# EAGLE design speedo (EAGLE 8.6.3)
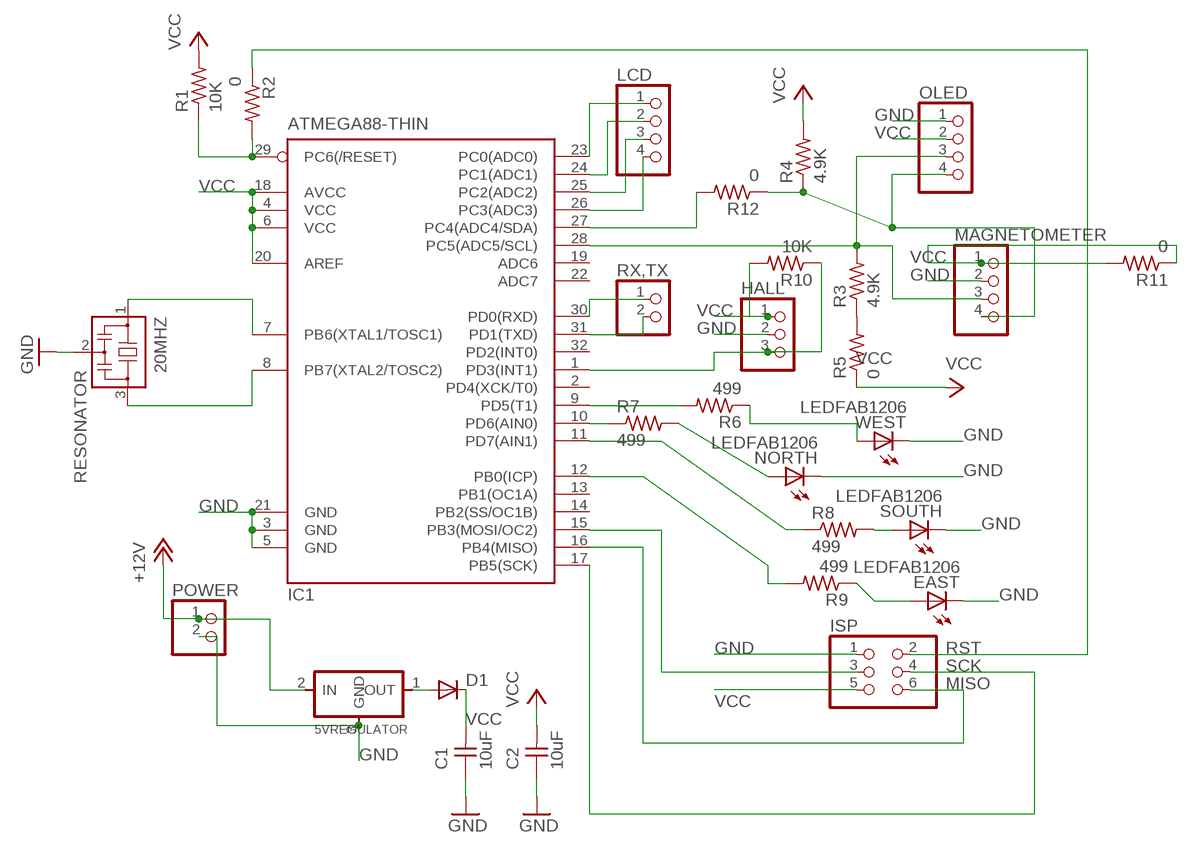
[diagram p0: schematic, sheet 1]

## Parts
5VREGULATOR  REGULATORSOT23  [SOT23]
20MHZ  RESONATOR  [EFOBM]
C1  10uF  CAP-UNPOLARIZEDFAB  [C1206FAB]
C2  10uF  CAP-UNPOLARIZEDFAB  [C1206FAB]
D1  DIODESOD123  [SOD123]
EAST  LEDFAB1206  [LED1206FAB]
HALL  PINHD-1X3  [1X03]
IC1  ATMEGA88-THIN  [TQFP32-08THIN]
ISP  PINHD-2X3-SMD  [2X03SMD]
LCD  PINHD-1X4  [1X04]
MAGNETOMETER  PINHD-1X4  [1X04]
NORTH  LEDFAB1206  [LED1206FAB]
OLED  PINHD-1X4  [1X04]
POWER  PINHD-1X2  [1X02]
R1  10K  RES-US1206FAB  [R1206FAB]
R2  0  RES-US1206FAB  [R1206FAB]
R3  4.9K  RES-US1206FAB  [R1206FAB]
R4  4.9K  RES-US1206FAB  [R1206FAB]
R5  0  RES-US1206FAB  [R1206FAB]
R6  499  RES-US1206FAB  [R1206FAB]
R7  499  RES-US1206FAB  [R1206FAB]
R8  499  RES-US1206FAB  [R1206FAB]
R9  499  RES-US1206FAB  [R1206FAB]
R10  10K  RES-US1206FAB  [R1206FAB]
R11  0  RES-US1206FAB  [R1206FAB]
R12  0  RES-US1206FAB  [R1206FAB]
RX,TX  PINHD-1X2  [1X02]
SOUTH  LEDFAB1206  [LED1206FAB]
WEST  LEDFAB1206  [LED1206FAB]

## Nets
+12V: 5VREGULATOR.2(IN) POWER.1
GND: 5VREGULATOR.3(GND) 20MHZ.2 C1.1 C2.1 EAST.2(C) HALL.2 IC1.3(GND) IC1.5(GND) IC1.21(GND) ISP.1 MAGNETOMETER.2 NORTH.2(C) OLED.1 POWER.2 SOUTH.2(C) WEST.2(C)
MISO: IC1.16(PB4(MISO)) ISP.6
N$1: IC1.29(PC6(/RESET)) R1.1 R2.2
N$2: 20MHZ.1 IC1.7(PB6(XTAL1/TOSC1))
N$3: 20MHZ.3 IC1.8(PB7(XTAL2/TOSC2))
N$4: 5VREGULATOR.1(OUT) D1.ANODE(A)
N$5: HALL.3 IC1.1(PD3(INT1)) R10.1
N$6: IC1.30(PD0(RXD)) RX,TX.1
N$7: MAGNETOMETER.4 OLED.4 R4.1 R12.1
N$8: IC1.28(PC5(ADC5/SCL)) MAGNETOMETER.3 OLED.3 R3.2
N$9: IC1.31(PD1(TXD)) RX,TX.2
N$10: IC1.27(PC4(ADC4/SDA)) R12.2
N$11: EAST.1(A) R9.1
N$12: IC1.9(PD5(T1)) R6.2
N$13: R6.1 WEST.1(A)
N$14: IC1.23(PC0(ADC0)) LCD.1
N$15: IC1.24(PC1(ADC1)) LCD.2
N$16: IC1.25(PC2(ADC2)) LCD.3
N$17: IC1.15(PB3(MOSI/OC2)) ISP.3
N$18: IC1.26(PC3(ADC3)) LCD.4
N$19: NORTH.1(A) R7.2
N$20: R8.2 SOUTH.1(A)
N$21: IC1.12(PB0(ICP)) R9.2
N$22: IC1.10(PD6(AIN0)) R7.1
N$23: IC1.11(PD7(AIN1)) R8.1
RST: ISP.2 R2.1
SCK: IC1.17(PB5(SCK)) ISP.4
VCC: C1.2 C2.2 D1.CATHODE(C) HALL.1 IC1.4(VCC) IC1.6(VCC) IC1.18(AVCC) IC1.20(AREF) ISP.5 MAGNETOMETER.1 OLED.2 R1.2 R3.1 R4.2 R5.1 R5.2 R10.2 R11.1 R11.2
Unconnected: IC1.2(PD4(XCK/T0)) IC1.13(PB1(OC1A)) IC1.14(PB2(SS/OC1B)) IC1.19(ADC6) IC1.22(ADC7) IC1.32(PD2(INT0))

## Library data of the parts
5VREGULATOR = fab:REGULATOR
20MHZ = fab:RESONATOR
C1 C2 = fab:CAP-UNPOLARIZED
D1 = fab:DIODE: DIODE
EAST NORTH SOUTH WEST = fab:LED: LED
HALL = pinhead:PINHD-1X3: PIN HEADER
IC1 = fab:ATMEGA88-THIN
ISP = fab:PINHD-2X3-SMD: PIN HEADER
LCD MAGNETOMETER OLED = pinhead:PINHD-1X4: PIN HEADER
POWER RX,TX = pinhead:PINHD-1X2: PIN HEADER
R1-R12 = fab:RES-US: Resistor (US Symbol)

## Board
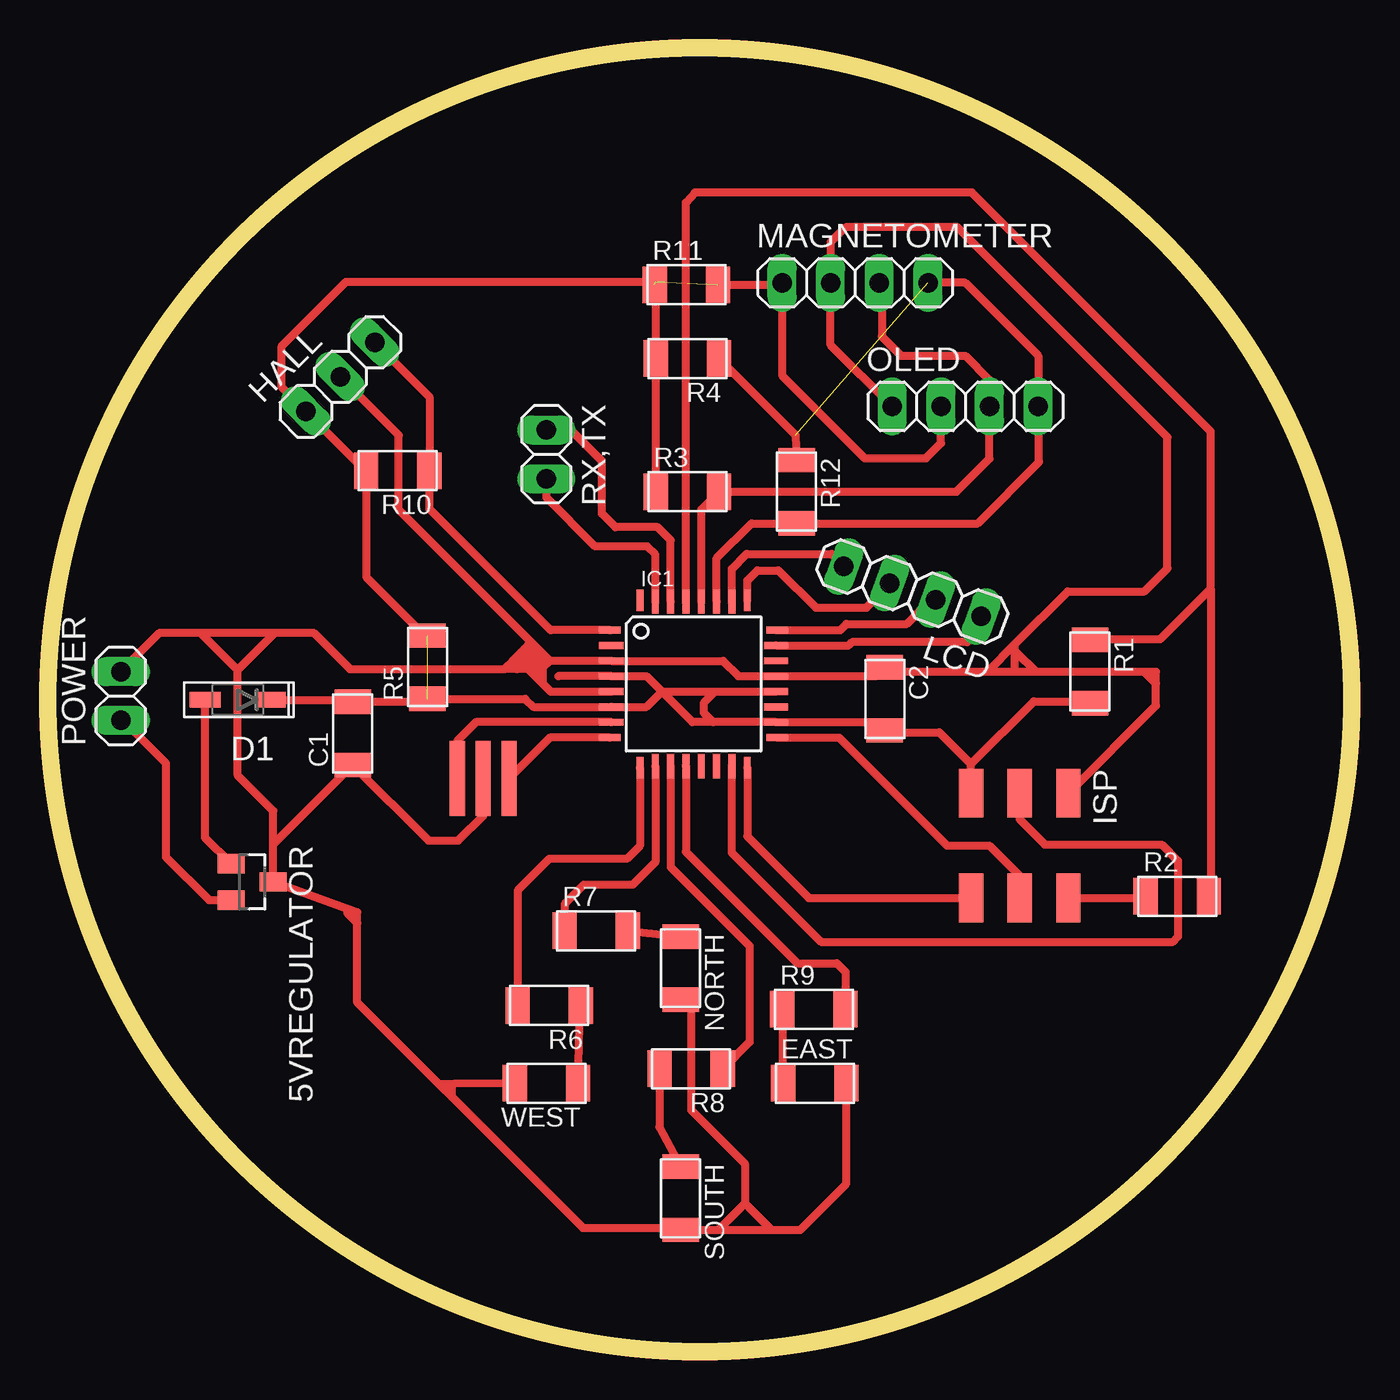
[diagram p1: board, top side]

Size 68 x 68 mm. Coordinates in mm from the lower left corner, seen from the top.
Outline: circle at 34,34 radius 34
Copper layers (1*16): Top 0.035mm / dielectric 1.5mm / Bottom 0.035mm
Design rules "default *": minimum track width 16mil, minimum drill 0.35mm, track to track 16mil, track to pad 16mil, pad to pad 16mil, via to via 16mil, smd to smd 16mil, copper to edge 40mil, drill to drill 6mil, minimum pad ring 10mil, minimum via ring 8mil, stop-mask expansion 4mil, vias tented up to drill 0mil, thermal gap 10mil

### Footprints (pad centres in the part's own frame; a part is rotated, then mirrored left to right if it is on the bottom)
SOT23 = smd 1 x 1.4: 1 -0.95,-1.1; 2 0.95,-1.1; 3 0,1.1
EFOBM = smd 0.8 x 3.9: 1 -1.35,0; 2 0,0; 3 1.35,0
C1206FAB = smd 1.27 x 1.905: 1 -1.651,0; 2 1.651,0
SOD123 = smd 1.6 x 0.8: ANODE 1.7,0; CATHODE -1.7,0
LED1206FAB = smd 1.27 x 1.905: 1 -1.651,0; 2 1.651,0
1X03 = drill 1.016 long: 1 -2.54,0; 2 0,0; 3 2.54,0
TQFP32-08THIN = smd 1.118 x 0.356: 1 -4.369,2.8; 8 -4.369,-2.8; 17 4.369,-2.8; 24 4.369,2.8 | smd 1.27 x 0.356: 2 -4.293,2; 3 -4.293,1.2; 4 -4.293,0.4; 5 -4.293,-0.4; 6 -4.293,-1.2; 7 -4.293,-2; 18 4.293,-2; 19 4.293,-1.2; 20 4.293,-0.4; 21 4.293,0.4; 22 4.293,1.2; 23 4.293,2 | smd 0.356 x 1.118: 9 -2.8,-4.369; 16 2.8,-4.369; 25 2.8,4.369; 32 -2.8,4.369 | smd 0.356 x 1.27: 10 -2,-4.293; 14 1.2,-4.293; 15 2,-4.293; 26 2,4.293; 27 1.2,4.293; 31 -2,4.293 | smd 0.35 x 1.27: 11 -1.2,-4.293; 12 -0.4,-4.293; 13 0.4,-4.293; 28 0.4,4.293; 29 -0.4,4.293; 30 -1.2,4.293
2X03SMD = smd 2.54 x 1.27: 1 -2.54,2.54; 2 2.92,2.54; 3 -2.54,0; 4 2.92,0; 5 -2.54,-2.54; 6 2.92,-2.54
1X04 = drill 1.016 long: 1 -3.81,0; 2 -1.27,0; 3 1.27,0; 4 3.81,0
1X02 = drill 1.016 long: 1 -1.27,0; 2 1.27,0
R1206FAB = smd 1.27 x 1.905: 1 -1.651,0; 2 1.651,0

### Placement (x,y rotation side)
5VREGULATOR  10.65,24.5 270 top
20MHZ  22.7,29.9 0 top
C1  15.9,32.25 90 top
C2  43.65,34.05 270 top
D1  9.9,34 180 top
EAST  40,14 0 top
HALL  15.25,50.85 45 top
IC1  33.68,34.83 0 top
ISP  50.69,26.58 270 top
LCD  45.1,39.65 160 top
MAGNETOMETER  42.1,55.75 0 top
NORTH  33,20 270 top
OLED  47.85,49.3 0 top
POWER  3.8,34.2 90 top
R1  54.35,35.47 270 top
R2  58.9,23.75 0 top
R3  33.35,44.85 0 top
R4  33.35,51.8 180 top
R5  19.8,35.7 90 top
R6  26.15,18.05 180 top
R7  28.6,21.95 0 top
R8  33.55,14.75 180 top
R9  39.95,17.85 0 top
R10  18.25,45.95 180 top
R11  33.3,55.65 0 top
R12  39.05,44.85 270 top
RX,TX  26,46.8 270 top
SOUTH  33,8 270 top
WEST  26,14 180 top

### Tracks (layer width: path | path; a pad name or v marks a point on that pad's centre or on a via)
+12V
  Top 0.406: POWER.1 3.92,32.93 6.15,30.7 6.15,25.8 8.4,23.55 5VREGULATOR.2
GND
  Top 0.406: 26.18,36.03 IC1.3 35.22,36.03 36.02,35.23 IC1.21 43.18,35.23 C2.1 | 26.18,36.03 25.8,35.65 | 25.8,35.65 25.8,34.85 | 25.8,34.85 26.22,34.43 IC1.5 | C2.1 43.85,35.5 | 15.62,23.1 16.14,22.91 16.14,22.35 | 15.62,23.1 5VREGULATOR.3 11.75,26.45 | 11.75,26.45 C1.1 | 11.75,26.45 11.75,28.2 9.9,30.05 9.9,35.55 | 16.1,30.8 C1.1 | C1.1 19.85,26.65 21.4,26.65 22.75,28 22.75,29.85 20MHZ.2 | 7.95,37.5 11.85,37.5 | 11.85,37.5 13.85,37.5 15.75,35.6 23.8,35.6 | 9.9,35.55 7.95,37.5 | 9.9,35.55 11.85,37.5 | 26.16,36.05 25.18,37.03 | 25.18,37.03 18.3,43.91 18.3,47.8 HALL.2 | 23.8,35.6 24.25,36.05 | 24.25,36.05 24.45,36.05 | 24.6,36.05 25.15,36.05 | 25.15,36.05 25.65,36.05 | 25.65,36.05 25.8,36.05 | 25.8,36.05 26.16,36.05 | 26.16,36.05 26.18,36.03 | 25.8,34.85 25.4,35.25 | 25.4,35.25 25.05,35.6 | 25.05,35.6 24.45,35.6 | 24.45,35.6 23.8,35.6 | 25.05,35.6 24.6,36.05 | 24.6,36.05 24.45,36.05 | 24.45,35.6 24.45,36.05 | 25.4,35.25 25.4,35.8 25.15,36.05 | 25.8,35.65 25.8,36.05 | OLED.1 40.83,52.51 MAGNETOMETER.2 40.83,57.88 41.6,58.65 47.45,58.65 58.4,47.7 58.4,40.85 57.2,39.65 53.2,39.65 50.45,36.9 | 20.4,13.95 16.14,18.21 16.14,22.35 | 20.4,13.95 21.07,13.28 | 21.07,13.28 27.9,6.45 33.1,6.45 SOUTH.2 37.73,6.35 | NORTH.2 33.55,18.05 33.55,12.6 36.35,9.8 36.35,7.73 | WEST.2 21.15,13.96 | 21.15,13.96 20.4,13.95 | EAST.2 41.65,8.75 39.25,6.35 37.73,6.35 | 36.35,7.73 35,6.38 | 24.25,36.05 24.68,36.48 | 24.68,36.48 24.85,36.65 | 24.85,36.65 25.18,36.98 25.18,37.03 | 25.65,36.05 25.05,36.65 24.85,36.65 | 25.15,36.05 24.73,36.48 24.68,36.48 | 57.8,34.85 57.8,33.69 ISP.1 | 57.8,34.85 57.8,35.45 57.2,35.45 | 57.2,35.45 51.55,35.45 | 51.55,35.45 50.45,35.45 | 50.45,35.45 49,35.45
  Top 0.406: 49,35.45 43.9,35.45 C2.1 | 50.45,35.45 50.45,36.55 | 50.45,36.55 50.45,36.9 | 7.95,37.5 5.83,37.5 POWER.2 | 36.35,7.73 37.73,6.35 | 50.45,36.9 49,35.45 | 50.45,36.55 51.55,35.45 | 57.2,35.45 57.8,34.85 | 15.62,23.1 15.62,22.87 16.14,22.35 | 21.07,13.28 21.07,13.89 21.15,13.96
MISO
  Top 0.406: IC1.16 36.48,26.87 39.69,23.66 ISP.6
N$1
  Top 0.406: IC1.29 33.28,59.93 33.75,60.45 48.2,60.45 60.65,48 60.65,39.8 | 60.65,39.8 58,37.15 54.32,37.15 R1.1 | 60.65,39.8 60.65,23.85 R2.2
N$2
  Top 0.406: IC1.7 22.33,32.83 21.35,31.85 20MHZ.1
N$3
  Top 0.406: IC1.8 26.18,32.03 20MHZ.3
N$4
  Top 0.406: 5VREGULATOR.1 8.2,26.8 D1.ANODE
N$5
  Top 0.406: HALL.3 19.9,49.79 R10.1 19.9,43.95 26.22,37.63 IC1.1
N$6
  Top 0.406: RX,TX.1 27.28,48.07 28.9,46.45 28.9,43.7 29.6,43 31.8,43 32.48,42.32 IC1.30
N$7  (1 unrouted)
  Top 0.406: MAGNETOMETER.4 47.85,55.75 51.66,51.94 OLED.4 | R4.1 39,47.8 R12.1
N$8
  Top 0.406: IC1.28 34.08,43.93 R3.2 47.4,44.85 49.12,46.57 OLED.3 49.12,50.68 47.85,51.95 44.5,51.95 43.5,52.95 43.5,55.62 MAGNETOMETER.3
N$9
  Top 0.406: IC1.31 31.68,41.57 31.25,42 28.55,42 26,44.55 RX,TX.2
N$10
  Top 0.406: IC1.27 34.88,41.38 36.7,43.2 R12.2 48.5,43.2 51.7,46.4 51.7,49.25
N$11
  Top 0.406: R9.1 EAST.1
N$12
  Top 0.406: IC1.9 30.88,26.38 30.2,25.7 26.15,25.7 24.5,24.05 R6.2
N$13
  Top 0.406: WEST.1 27.75,18 R6.1
N$14
  Top 0.406: IC1.23 41.78,36.83 41.95,37 47.95,37 47.95,37.62 LCD.1
N$15
  Top 0.406: IC1.24 41.33,37.63 41.65,37.95 44.8,37.95 46.07,39.22 LCD.2
N$16
  Top 0.406: IC1.25 36.48,40.23 37,40.75 38.1,40.75 40.05,38.8 42.7,38.8 43.91,40.01 LCD.3
N$17
  Top 0.406: ISP.3 50.69,27.76 52,26.45 58.1,26.45 58.95,25.6 58.95,21.65 58.65,21.35 40.35,21.35 35.68,26.02 IC1.15
N$18
  Top 0.406: IC1.26 35.68,40.83 36.45,41.6 40.87,41.6 LCD.4
N$19
  Top 0.406: R7.2 NORTH.1
N$20
  Top 0.406: R8.2 31.9,11.7 SOUTH.1
N$21
  Top 0.406: IC1.12 33.28,26.07 39.1,20.25 41.15,20.25 41.6,19.8 R9.2
N$22
  Top 0.406: IC1.10 31.68,25.53 30.5,24.35 27.95,24.35 26.95,23.35 R7.1
N$23
  Top 0.406: IC1.11 32.48,25.27 36.6,21.15 36.6,16.15 R8.1
RST
  Top 0.406: ISP.2 57.16,23.66 R2.1
SCK
  Top 0.406: IC1.17 41.27,32.03 46.9,26.4 49.1,26.4 50.69,24.81 ISP.4
VCC  (3 unrouted)
  Top 0.406: 26.62,35.23 IC1.4 31.22,35.23 32.02,34.43 | 32.02,34.43 34.8,34.43 | 34.8,34.43 IC1.20 | 32.02,34.43 31.22,33.63 IC1.6 25.32,33.63 24.9,34.05 R5.1 19.65,33.9 C1.2 15.8,34 D1.CATHODE | 34.7,32.83 IC1.18 43.02,32.83 43.65,32.2 C2.2 | 34.7,32.83 33.62,32.83 32.02,34.43 | 34.8,34.43 34.2,33.83 34.2,33.33 34.7,32.83 | C2.2 43.75,32.3 46.5,32.3 48.15,30.65 | 43.6,32.35 C2.2 | R5.2 19.65,37.35 16.6,40.4 R10.2 16.56,45.95 HALL.1 12.2,50.31 12.2,52.45 15.55,55.8 31.7,55.8 R4.2 | R11.2 38.19,55.65 MAGNETOMETER.1 38.29,50.91 42.6,46.6 45.8,46.6 46.58,47.38 OLED.2 46.35,49.07 | R4.2 R3.1 | ISP.5 48.15,30.65 | 31.8,51.9 R4.2 | 48.15,30.65 51.42,33.92 54.25,33.92 R1.2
